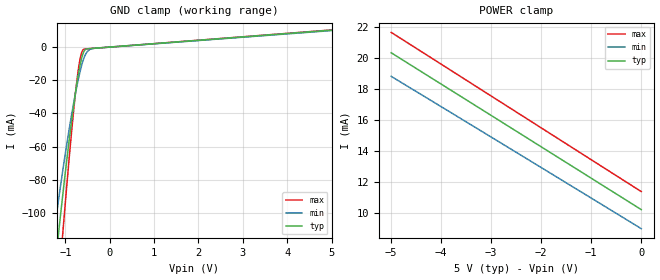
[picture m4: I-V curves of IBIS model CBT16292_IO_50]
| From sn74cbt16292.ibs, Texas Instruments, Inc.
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[Model]   CBT16292_IO_50
Model_type  Terminator
| variable   typ   min   max
C_comp   3.70pF   2.78pF   7.69pF
| C_tri-state   3.70pF   2.78pF   7.69pF
[Temperature Range]   40   100   -40
| Ambient temperature   25   85   -40
[Voltage range]   5   4.5   5.5
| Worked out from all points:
|   GND clamp passes 1 mA (typ) near -0.47 V on its own axis
[GND Clamp]
| CBT16292_IO_50
|   Voltage   I(typ)   I(min)   I(max)
-5V       -3.009A    -3.129A    -2.666A
-1.315V   -153.7mA   -123.9mA   -199.8mA
-1.225V   -130.2mA   -105.7mA   -168.2mA
-1.135V   -107.5mA   -88.38mA   -137.5mA
-1.055V   -88.09mA   -73.63mA   -110.9mA
-905mV    -54.02mA   -47.91mA   -63.96mA
-770mV    -27.05mA   -27.52mA   -26.95mA
-670mV    -11.04mA   -14.87mA   -7.274mA
-585mV    -2.724mA   -6.783mA   -1.27mA
-505mV    -1.106mA   -2.677mA   -1.046mA
-360mV    -735uA     -766.5uA   -743.7uA
5V        10.19mA    9.945mA    10.33mA
[POWER Clamp]
| CBT16292_IO_50
|   Voltage   I(typ)   I(min)   I(max)
-5V       20.35mA    18.82mA    21.67mA
-3.725V   17.76mA    16.32mA    19.04mA
-2.59V    15.46mA    14.08mA    16.7mA
-84.45fV  10.19mA    8.953mA    11.36mA
